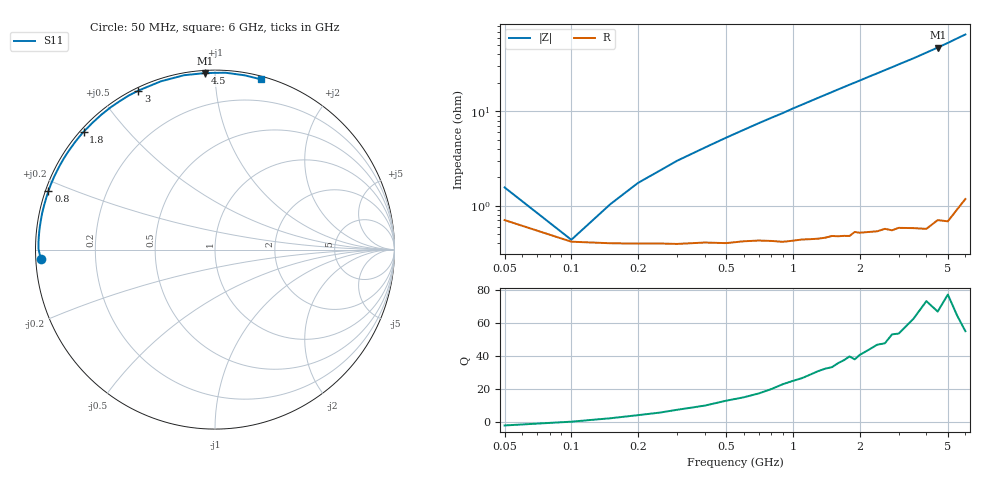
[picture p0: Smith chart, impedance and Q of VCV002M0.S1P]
! Infineon Technologies  Discrete & RF Semiconductors
! BBY 56-03
! Si Tuning Diode in SOD323
! VR =
! S-Parameters:  June  1999
# GHz  S  MA  R  50
!  f  S11
! GHz  MAG  ANG
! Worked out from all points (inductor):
!   34 points, 50 MHz to 6 GHz, reference 50 ohm
!   read as one part to ground: L = 1.47 nH near 200 MHz
!   highest Q = 73.5 at 4.5 GHz (marker M1), where L = 1.68 nH
!   S11 on the Smith chart (normalised r, x): 50 MHz: 0.01, -0.03; 800 MHz: 0.01, +0.17; 1.8 GHz: 0.01, +0.38; 3 GHz: 0.01, +0.63; 4.5 GHz: 0.01, +0.95; 6 GHz: 0.02, +1.30
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0.05  0.9722 -176.8
0.1  0.9835 179.7
0.15  0.9841 177.8
0.2  0.9842 176.1
0.25  0.9842 174.7
0.3  0.9844 173.2
0.5  0.9842 168.0
0.7  0.9834 163.0
0.8  0.9836 160.6
0.9  0.9841 158.3
1  0.9838 155.8
1.2  0.9835 151.2
1.3  0.9835 148.9
1.4  0.9833 146.7
1.6  0.9831 142.3
1.8  0.9834 138.1
2  0.9826 134.1
2.2  0.9828 130.1
2.4  0.983 126.4
2.6  0.9826 122.7
2.8  0.9838 119.2
3  0.9834 115.7
3.5  0.985 107.8
4  0.9867 100.1
4.5  0.9852 93.1
5  0.9872 86.6
5.5  0.9849 80.4
6  0.9827 75.0
